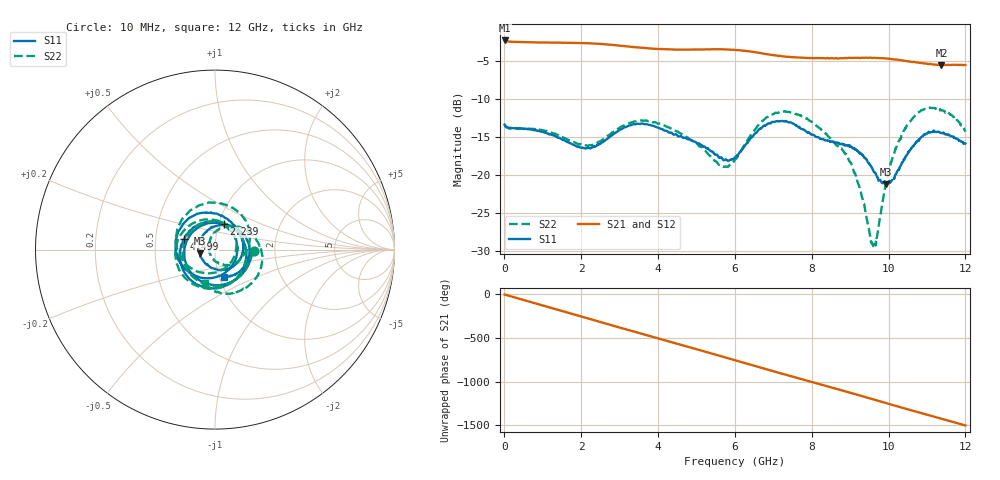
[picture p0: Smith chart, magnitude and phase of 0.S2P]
!Agilent Technologies,E5071C,MY46316741,A.11.02
!Date: Wed Sep 16 11:41:56 2020
!Data & Calibration Information:
!Freq	S11:SOLT2(ON)	S21:SOLT2(ON)	S12:SOLT2(ON)	S22:SOLT2(ON)
!PortZ  Port1:50+j0  Port2:50+j0
!Above PortZ is port z conversion or system Z0 setting when saving the data.
!When reading, reference impedance value at option line is always used.
# Hz S dB R 50
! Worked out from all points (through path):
!   1561 points, 10 MHz to 12 GHz, reference 50 ohm
!   highest |S21| = -2.22 dB at 10 MHz (marker M1); lowest = -5.5 dB at 11.38 GHz (marker M2)
!   group delay of S21, straight-line fit = 347 ps
!   lowest |S11| = -21.2 dB at 9.94 GHz (marker M3), VSWR 1.19, Z = 42.2 - j1.75 ohm
!   |S11| at or under -10 dB: start of sweep to end of sweep
!   |S22| runs from -29.4 to -11.1 dB; largest |S21 - S12| = 0.0053
!   S11 on the Smith chart (normalised r, x): 10 MHz: 1.55, -0.03; 2.239 GHz: 1.06, +0.31; 4.499 GHz: 0.70, +0.08; 12 GHz: 1.06, -0.33
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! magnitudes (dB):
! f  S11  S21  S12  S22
! 10 MHz  -13.3  -2.2  -2.2  -13.3
! 2.016 GHz  -16.4  -2.6  -2.6  -16.0
! 2.239 GHz  -16.5  -2.6  -2.6  -16.0
! 3.284 GHz  -13.4  -3.1  -3.1  -13.1
! 4.007 GHz  -13.7  -3.4  -3.4  -13.2
! 4.499 GHz  -14.7  -3.4  -3.4  -14.2
! 5.651 GHz  -17.7  -3.4  -3.4  -18.7
! 6.005 GHz  -17.6  -3.5  -3.5  -17.9
! 6.935 GHz  -13.1  -4.1  -4.1  -12.0
! 7.396 GHz  -13.0  -4.4  -4.4  -11.6
! 8.011 GHz  -14.7  -4.5  -4.5  -13.0
! 8.987 GHz  -16.0  -4.5  -4.5  -18.2
! 9.279 GHz  -17.2  -4.5  -4.5  -22.3
! 9.594 GHz  -19.4  -4.5  -4.5  -29.1
! 9.694 GHz  -20.1  -4.5  -4.6  -28.2
! 9.94 GHz  -21.2  -4.6  -4.6  -21.0
! 10 GHz  -21.0  -4.6  -4.7  -19.6
! 10.23 GHz  -19.4  -4.8  -4.8  -15.9
! 10.58 GHz  -16.5  -5.0  -5.0  -12.8
! 10.97 GHz  -14.6  -5.3  -5.3  -11.2
! 11.38 GHz  -14.4  -5.5  -5.5  -11.4
! 12 GHz  -15.8  -5.5  -5.5  -14.2
